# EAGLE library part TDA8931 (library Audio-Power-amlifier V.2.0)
The TDA8931 is a switching power stage for high efficiency class-D audio power amplifier systems. It contains a Single-Ended (SE) power stage, drive logic, protection control logic, a full differential input comparator and a HVP charger to charge the SE capacitor. With this amplifier a compact 1 ´ 20 W closed loop self-oscillating digital amplifier system can be built. The TDA8931 has a high efficiency so that a heat sink is not required up to 20 W (RMS). The system operates on an asymmetrical and a symmetrical supply voltage.
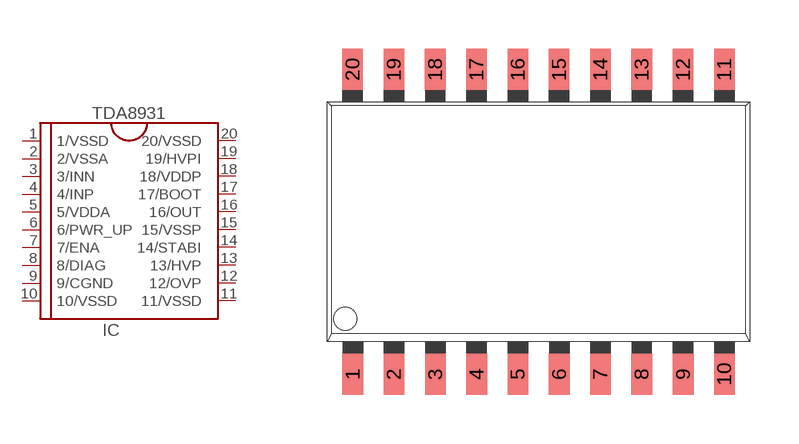
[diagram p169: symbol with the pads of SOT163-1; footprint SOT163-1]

Designator prefix IC

## TDA8931  [SOT163-1]
1  1/VSSD  pwr
2  2/VSSA  pwr
3  3/INN  in
4  4/INP  in
5  5/VDDA  pwr
6  6/PWR_UP  in
7  7/ENA  in
8  8/DIAG  out
9  9/CGND  pwr
10  10/VSSD  pwr
11  11/VSSD  pwr
12  12/OVP  in
13  13/HVP  out
14  14/STABI
15  15/VSSP  pwr
16  16/OUT  out
17  17/BOOT
18  18/VDDP  pwr
19  19/HVPI  out
20  20/VSSD  pwr

## Footprint SOT163-1 (pad centres in mm)
smd 0.635 x 1.27: 1 -5.71,-4.685; 2 -4.445,-4.685; 3 -3.17,-4.685; 4 -1.9,-4.685; 5 -0.635,-4.685; 6 0.64,-4.685; 7 1.905,-4.685; 8 3.175,-4.685; 9 4.45,-4.685; 10 5.715,-4.685; 11 5.715,4.685; 12 4.445,4.685; 13 3.175,4.685; 14 1.905,4.685; 15 0.635,4.685; 16 -0.635,4.685; 17 -1.905,4.685; 18 -3.175,4.685; 19 -4.445,4.685; 20 -5.715,4.685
